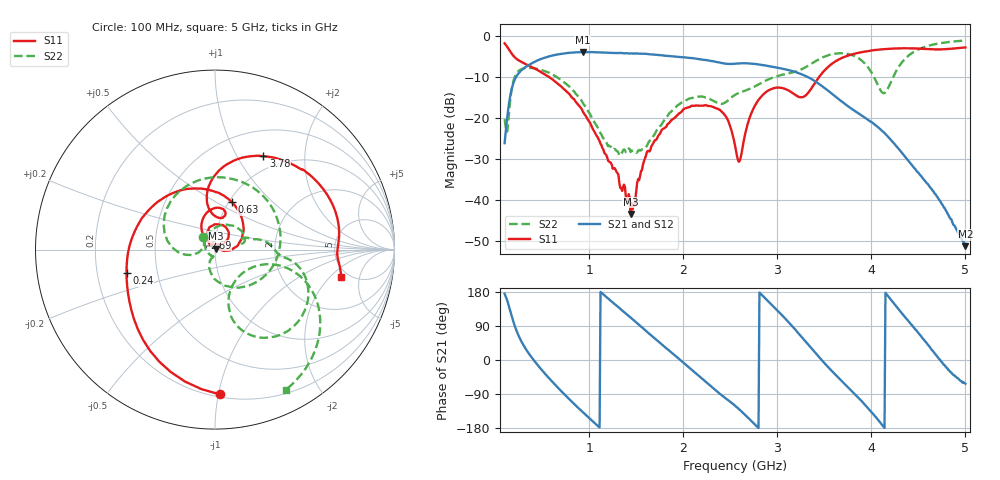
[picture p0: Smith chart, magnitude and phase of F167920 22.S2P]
!  2-Port S-parameters saved by WinCal
! VAR MeasName=S-Parameters (CALIBRATED_DATA) read from VNA (N5242A)
! VAR MeasDate=2016-11-22 9:56:15
! VAR NAME=F167920 22
! VAR FILENAME=F167920 22.S2P
! VAR DATE=2016-11-22 9:56:15
! VAR PHYS_PORTS=1,2
# Hz S DB R 50
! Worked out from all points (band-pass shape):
!   491 points, 100 MHz to 5 GHz, reference 50 ohm
!   highest |S21| = -3.96 dB at 930 MHz (marker M1); lowest = -51.2 dB at 5 GHz (marker M2)
!   |S21| within 3 dB of the highest: 369.1 MHz to 2.795 GHz (2.426 GHz wide, 153 % of centre)
!   lowest |S11| = -43.3 dB at 1.44 GHz (marker M3), VSWR 1.01, Z = 50.3 + j0.615 ohm
!   |S11| at or under -10 dB: 571.9 MHz to 3.445 GHz (2.873 GHz wide, 143 % of centre)
!   |S22| runs from -29.2 to -1.2 dB; largest |S21 - S12| = 0.00087
!   S11 on the Smith chart (normalised r, x): 100 MHz: 0.22, -1.01; 240 MHz: 0.33, -0.12; 630 MHz: 1.03, +0.60; 2.69 GHz: 0.88, +0.12; 3.78 GHz: 0.82, +1.29; 5 GHz: 4.30, -2.75
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1e8  -1.86 -88.0  -26.13 174.9  -26.12 175.1  -20.28 135.0
2.4e8  -5.85 -165.3  -9.39 69.1  -9.39 69.1  -8.76 132.7
4.3e8  -8.11 126.7  -6.23 -6.7  -6.23 -6.8  -7.98 43.4
6.3e8  -11.00 70.8  -4.69 -63.5  -4.70 -63.5  -9.71 -20.8
9.2e8  -17.81 10.0  -3.98 -134.9  -3.98 -134.9  -15.82 -92.0
9.3e8  -18.36 8.0  -3.96 -137.5  -3.96 -137.5  -16.30 -93.8
1.17e9  -28.74 -2.8  -4.12 168.8  -4.12 168.8  -25.62 -110.6
1.44e9  -43.32 63.5  -4.30 112.0  -4.30 112.0  -28.28 -116.4
1.74e9  -24.10 128.9  -4.70 47.9  -4.70 47.8  -22.35 133.8
1.99e9  -18.24 106.6  -5.24 -4.3  -5.23 -4.4  -16.18 62.4
2.25e9  -16.98 70.3  -5.95 -60.2  -5.95 -60.2  -15.12 18.3
2.45e9  -19.55 44.0  -6.81 -101.0  -6.81 -101.0  -16.18 20.4
2.55e9  -26.65 42.4  -6.80 -120.4  -6.81 -120.4  -14.39 20.3
2.6e9  -30.41 92.6  -6.72 -131.3  -6.72 -131.3  -13.85 17.7
2.69e9  -21.03 130.3  -6.72 -152.7  -6.72 -152.8  -13.07 15.0
3.07e9  -12.82 78.0  -8.10 113.1  -8.11 113.0  -9.40 -1.4
3.37e9  -12.51 98.8  -10.61 28.6  -10.62 28.5  -6.70 -10.4
3.78e9  -4.64 62.6  -17.61 -78.7  -17.63 -78.7  -4.60 -55.2
4.01e9  -3.56 41.7  -21.16 -139.6  -21.20 -139.5  -9.26 -76.6
4.19e9  -3.18 27.7  -24.85 164.9  -24.89 165.0  -12.15 -21.8
4.5e9  -3.13 7.4  -33.32 71.2  -33.35 71.6  -3.34 -31.2
5e9  -2.86 -12.4  -51.17 -62.7  -50.82 -62.9  -1.15 -63.3
